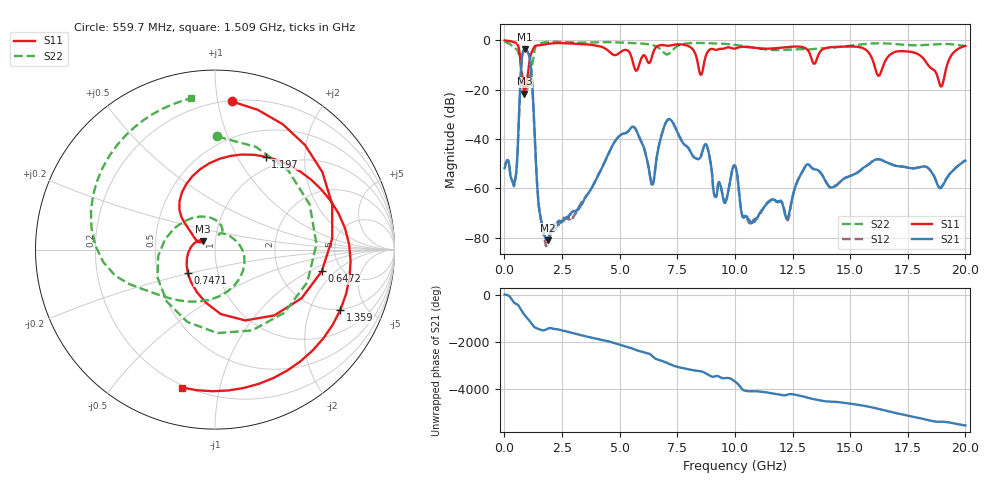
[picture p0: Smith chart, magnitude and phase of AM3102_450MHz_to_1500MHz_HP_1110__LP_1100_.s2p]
!Agilent Technologies,E8364B,MY43040894,A.07.50.67
!Agilent E8364B: A.07.50.67
!Date: Thursday, January 11, 2018 06:45:29
!Correction: S11(Full 2 Port(1,2))
!S21(Full 2 Port(1,2))
!S12(Full 2 Port(1,2))
!S22(Full 2 Port(1,2))
!S2P File: Measurements: S11, S21, S12, S22:
# Hz S  dB  R 50
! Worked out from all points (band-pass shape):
!   1601 points, 10 MHz to 20 GHz, reference 50 ohm
!   highest |S21| = -3.66 dB at 897.1 MHz (marker M1); lowest = -81.0 dB at 1.897 GHz (marker M2)
!   |S21| within 3 dB of the highest: 770 MHz to 1.089 GHz (319 MHz wide, 34.3 % of centre)
!   lowest |S11| = -21.6 dB at 872.1 MHz (marker M3), VSWR 1.18, Z = 43.4 + j3.97 ohm
!   |S11| at or under -10 dB: 706.1 MHz to 1.066 GHz (360.4 MHz wide, 40.7 % of centre); 16.05 GHz to 16.45 GHz (402.7 MHz wide, 2.48 % of centre); 18.38 GHz to 19.21 GHz (832.5 MHz wide, 4.43 % of centre)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
!   |S22| runs from -21.3 to -0.5 dB; largest |S21 - S12| = 0.0018
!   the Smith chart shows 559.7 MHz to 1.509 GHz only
!   S11 on the Smith chart (normalised r, x): 559.7 MHz: 0.21, +1.10; 647.2 MHz: 3.53, -1.35; 747.1 MHz: 0.72, -0.20; 1.197 GHz: 0.83, +1.32; 1.359 GHz: 1.95, -3.29; 1.509 GHz: 0.19, -0.77
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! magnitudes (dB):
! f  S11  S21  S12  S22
! 10 MHz  -0.1  -51.9  -50.5  -0.5
! 559.7 MHz  -1.6  -47.6  -47.7  -4.0
! 647.2 MHz  -4.3  -27.2  -27.3  -6.1
! 747.1 MHz  -14.0  -8.7  -8.7  -12.6
! 872.1 MHz  -21.6  -3.7  -3.7  -20.1
! 897.1 MHz  -21.1  -3.7  -3.7  -21.2
! 1.197 GHz  -4.6  -16.4  -16.4  -10.4
! 1.359 GHz  -2.2  -47.9  -47.8  -2.6
! 1.509 GHz  -2.0  -68.4  -68.2  -1.4
! 1.897 GHz  -1.5  -81.0  -80.7  -0.7
! 3.346 GHz  -1.6  -66.6  -65.7  -1.0
! 5.032 GHz  -4.8  -38.5  -38.5  -0.9
! 6.407 GHz  -6.5  -58.5  -58.5  -1.9
! 6.682 GHz  -2.2  -43.6  -43.7  -3.0
! 8.743 GHz  -6.2  -42.2  -42.2  -1.2
! 9.568 GHz  -3.3  -66.0  -64.9  -1.5
! 10.01 GHz  -3.4  -50.9  -50.9  -1.9
! 10.67 GHz  -2.9  -73.6  -74.3  -2.8
! 13.34 GHz  -8.0  -51.8  -51.7  -3.6
! 16.68 GHz  -6.4  -49.8  -49.8  -1.4
! 18.95 GHz  -18.7  -59.8  -59.6  -1.5
! 20 GHz  -2.3  -48.8  -48.7  -2.3
